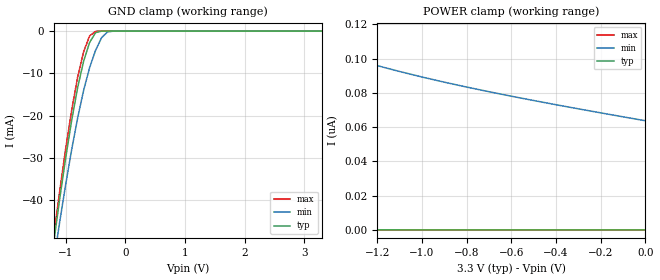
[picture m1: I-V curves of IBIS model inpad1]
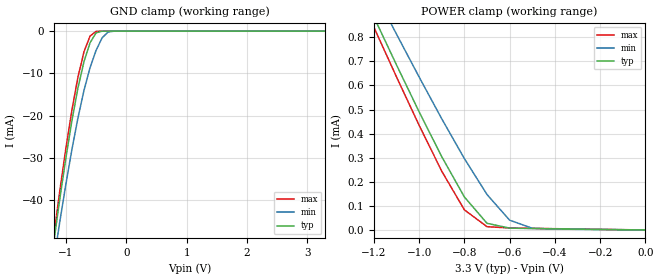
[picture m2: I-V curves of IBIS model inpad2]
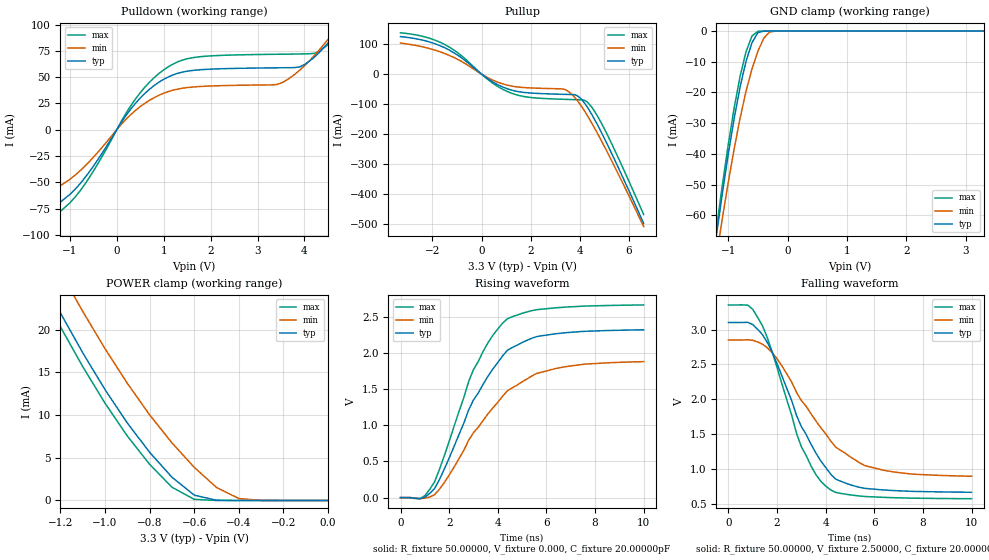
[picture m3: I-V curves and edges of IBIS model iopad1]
| IBIS file 71650da.ibs created by s2ibis2 version 1.2
| North Carolina State University Electronics Research Laboratory  1995
[IBIS ver]   2.1
[File name]   71650da.ibs
[File Rev]   1.2
[Date]   11/10/2004
[Source]   Integrated Device Technology, Inc.
[Notes]   1.Temperatures: typ=25C, min=100C, max=0C
   2.Ramp rates based on 50 ohm load.
   3.The model for the open-drain dta pin does not reflect a
   pulsed pull-up device which aides the output on highz.
[Disclaimer] Integrated Device Technology, Inc. ("IDT") hereby grants the
   user of this IBIS model a non-exclusive, nontransferable
   license to use this IBIS model under the following terms. The
   user is granted this license only to use the IBIS model and is
   not granted rights to sell, copy (except as needed to run the
   IBIS model), rent, lease or sub-license the IBIS model in
   whole or in part, or in modified form to anyone. The User may
   modify the IBIS model to suit its specific applications, but
   rights to derivative works and such modifications shall belong
   to IDT. This IBIS model is provided on an AS IS" basis and IDT
   makes absolutely no warranty with respect to the information
   contained herein. IDT DISCLAIMS AND CUSTOMER WAIVES ALL
   WARRANTIES, EXPRESS AND IMPLIED, INCLUDING WARRANTIES OF
   MERCHANTABILITY AND FITNESS FOR A PARTICULAR PURPOSE. THE
   ENTIRE RISK AS TO QUALITY AND PERFORMANCE IS WITH THE USER
   ACCORDINGLY, IN NO EVENT SHALL IDT BE LIABLE FOR ANY DIRECT OR
   INDIRECT DAMAGES, WHETHER IN CONTRACT OR TORT, INCLUDING ANY
   LOST PROFITS OR OTHER INCIDENTAL, CONSEQUENTIAL, EXEMPLARY, OR
   PUNITIVE DAMAGES ARISING OUT OF THE USE OR APPLICATION OF THE
   IBIS model. Further, IDT reserves the right to make changes
   without notice to any product herein to improve reliability,
   function, or design. IDT does not convey any license under
   patent rights or any other intellectual property rights,
   including those of third parties. IDT is not obligated to
   provide maintenance or support for the licensed IBIS model.
[Copyright]   Copyright 2001, Integrated Device Technology, Inc. all rights
   reserved
|   Component 72v71650
[Component]   72v71650
[Manufacturer]   Integrated Device Technology
[Package]
| DA144
| variable   typ   min   max
R_pkg   51.20m   43.90m   58.40m
L_pkg   4.19nH   3.49nH   4.89nH
C_pkg   0.81pF   0.74pF   0.87pF
[Pin]   signal_name   model_name   R_pin   L_pin   C_pin
143   ode   inpad1
144   resetx   inpad1
2   clk   inpad1
3   foi   inpad1
4   fe_hclk   inpad1
5   wfps   inpad1
6   tms   inpad2
7   tdi   inpad2
8   tdo   iopad1
9   tck   inpad1
10   trstx   inpad2
11   dsx   inpad1
12   csx   inpad1
13   rwx   inpad1
15   a0   inpad1
16   a1   inpad1
17   a2   inpad1
18   a3   inpad1
19   a4   inpad1
20   a5   inpad1
21   a6   inpad1
22   a7   inpad1
23   a8   inpad1
24   a9   inpad1
25   a10   inpad1
26   a11   inpad1
27   a12   inpad1
28   a13   inpad1
29   a14   inpad1
32   dtax   outpad3
35   d15   iopad2
36   d14   iopad2
37   d13   iopad2
38   d12   iopad2
41   d11   iopad2
42   d10   iopad2
43   d9   iopad2
44   d8   iopad2
47   d7   iopad2
48   d6   iopad2
49   d5   iopad2
50   d4   iopad2
53   d3   iopad2
54   d2   iopad2
55   d1   iopad2
56   d0   iopad2
59   rx31   inpad1
60   rx30   inpad1
61   rx29   inpad1
62   rx28   inpad1
63   rx27   inpad1
64   rx26   inpad1
65   rx25   inpad1
66   rx24   inpad1
93   rx23   inpad1
94   rx22   inpad1
95   rx21   inpad1
96   rx20   inpad1
97   rx19   inpad1
98   rx18   inpad1
99   rx17   inpad1
100   rx16   inpad1
101   rx15   inpad1
102   rx14   inpad1
103   rx13   inpad1
104   rx12   inpad1
105   rx11   inpad1
106   rx10   inpad1
107   rx9   inpad1
108   rx8   inpad1
135   rx7   inpad1
136   rx6   inpad1
137   rx5   inpad1
138   rx4   inpad1
139   rx3   inpad1
140   rx2   inpad1
141   rx1   inpad1
142   rx0   inpad1
69   tx31   iopad1
70   tx30   iopad1
71   tx29   iopad1
72   tx28   iopad1
75   tx27   iopad1
76   tx26   iopad1
77   tx25   iopad1
78   tx24   iopad1
81   tx23   iopad1
82   tx22   iopad1
83   tx21   iopad1
84   tx20   iopad1
87   tx19   iopad1
88   tx18   iopad1
89   tx17   iopad1
90   tx16   iopad1
111   tx15   iopad1
112   tx14   iopad1
113   tx13   iopad1
114   tx12   iopad1
117   tx11   iopad1
118   tx10   iopad1
119   tx9   iopad1
120   tx8   iopad1
123   tx7   iopad1
124   tx6   iopad1
125   tx5   iopad1
126   tx4   iopad1
129   tx3   iopad1
130   tx2   iopad1
131   tx1   iopad1
132   tx0   iopad1
110   vdd   POWER
116   vdd   POWER
122   vdd   POWER
128   vdd   POWER
134   vdd   POWER
14   vdd   POWER
33   vdd   POWER
39   vdd   POWER
45   vdd   POWER
51   vdd   POWER
57   vdd   POWER
67   vdd   POWER
73   vdd   POWER
79   vdd   POWER
85   vdd   POWER
91   vdd   POWER
109   vss   GND
115   vss   GND
121   vss   GND
127   vss   GND
133   vss   GND
1   vss   GND
34   vss   GND
40   vss   GND
46   vss   GND
52   vss   GND
58   vss   GND
68   vss   GND
74   vss   GND
80   vss   GND
86   vss   GND
92   vss   GND
| in   in   dummy_model
| oe   oe   dummy_model
[Pin Mapping]  pulldown_ref   pullup_ref   gnd_clamp_ref   power_clamp_ref
143   vss   vdd
144   vss   vdd
2   vss   vdd
3   vss   vdd
4   vss   vdd
5   vss   vdd
6   vss   vdd
7   vss   vdd
8   vss   vdd
9   vss   vdd
10   vss   vdd
11   vss   vdd
12   vss   vdd
13   vss   vdd
15   vss   vdd
16   vss   vdd
17   vss   vdd
18   vss   vdd
19   vss   vdd
20   vss   vdd
21   vss   vdd
22   vss   vdd
23   vss   vdd
24   vss   vdd
25   vss   vdd
26   vss   vdd
27   vss   vdd
28   vss   vdd
29   vss   vdd
32   vss   vdd
35   vss   vdd
36   vss   vdd
37   vss   vdd
38   vss   vdd
41   vss   vdd
42   vss   vdd
43   vss   vdd
44   vss   vdd
47   vss   vdd
48   vss   vdd
49   vss   vdd
50   vss   vdd
53   vss   vdd
54   vss   vdd
55   vss   vdd
56   vss   vdd
59   vss   vdd
60   vss   vdd
61   vss   vdd
62   vss   vdd
63   vss   vdd
64   vss   vdd
65   vss   vdd
66   vss   vdd
93   vss   vdd
94   vss   vdd
95   vss   vdd
96   vss   vdd
97   vss   vdd
98   vss   vdd
99   vss   vdd
100   vss   vdd
101   vss   vdd
102   vss   vdd
103   vss   vdd
104   vss   vdd
105   vss   vdd
106   vss   vdd
107   vss   vdd
108   vss   vdd
135   vss   vdd
136   vss   vdd
137   vss   vdd
138   vss   vdd
139   vss   vdd
140   vss   vdd
141   vss   vdd
142   vss   vdd
69   vss   vdd
70   vss   vdd
71   vss   vdd
72   vss   vdd
75   vss   vdd
76   vss   vdd
77   vss   vdd
78   vss   vdd
81   vss   vdd
82   vss   vdd
83   vss   vdd
84   vss   vdd
87   vss   vdd
88   vss   vdd
89   vss   vdd
90   vss   vdd
111   vss   vdd
112   vss   vdd
113   vss   vdd
114   vss   vdd
117   vss   vdd
118   vss   vdd
119   vss   vdd
120   vss   vdd
123   vss   vdd
124   vss   vdd
125   vss   vdd
126   vss   vdd
129   vss   vdd
130   vss   vdd
131   vss   vdd
132   vss   vdd
110   nc   vdd
116   nc   vdd
122   nc   vdd
128   nc   vdd
134   nc   vdd
14   nc   vdd
33   nc   vdd
39   nc   vdd
45   nc   vdd
51   nc   vdd
57   nc   vdd
67   nc   vdd
73   nc   vdd
79   nc   vdd
85   nc   vdd
91   nc   vdd
109   vss   nc
115   vss   nc
121   vss   nc
127   vss   nc
133   vss   nc
1   vss   nc
34   vss   nc
40   vss   nc
46   vss   nc
52   vss   nc
58   vss   nc
68   vss   nc
74   vss   nc
80   vss   nc
86   vss   nc
92   vss   nc
| Models and submodels in the file (5): inpad1 (Input), inpad2 (Input), iopad1 (3-state), iopad2 (3-state), outpad3 (Open_drain)
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|   Model inpad1
[Model]   inpad1
Model_type   Input
Polarity   Non-Inverting
Vinl =  0.80000V
Vinh =  2.00000V
|Vmeas =  1.50000V
C_comp   5.00000pF   NA   NA
[Temperature Range]   25.00000   100.00000   0.000
[Voltage Range]   3.30000V   3.00000V   3.60000V
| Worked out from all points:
|   GND clamp passes 1 mA (typ) near -0.53 V on its own axis
[GND_clamp]
| voltage   I(typ)   I(min)   I(max)
-3.3V     -310mA     -295.4mA   -315.4mA
-1.2V     -49.78mA   -54.27mA   -48.33mA
-1.1V     -39.5mA    -44.95mA   -37.65mA
-900mV    -21.04mA   -27.95mA   -18.63mA
-800mV    -13.32mA   -20.5mA    -10.85mA
-700mV    -7.09mA    -13.99mA   -4.876mA
-600mV    -2.698mA   -8.653mA   -1.161mA
-500mV    -374.6uA   -4.55mA    -53.22uA
-400mV    -11.83uA   -1.585mA   -1.231uA
-300mV    -285.2nA   -196.8uA   -25.38nA
-200mV    -6.527nA   -10.13uA   -459.3pA
3.3V      26.9pA     70.7nA     2.066pA
[POWER_clamp]
| voltage   I(typ)   I(min)   I(max)
-3.3V     3.879nA    456nA      684.6pA
-3V       2.36nA     327.1nA    413.6pA
-2.7V     1.415nA    242.1nA    246pA
-1.7V     242.2pA    118.8nA    39.53pA
-1.6V     203.7pA    113.3nA    32.78pA
-1.5V     171.8pA    108.3nA    27.21pA
-1.3V     123.7pA    99.68nA    18.83pA
-1.2V     105.8pA    95.94nA    15.74pA
-1V       78.71pA    89.29nA    11.07pA
-800mV    60.2pA     83.42nA    7.956pA
-600mV    47.4pA     78.08nA    5.874pA
0V        26.91pA    63.75nA    2.762pA
|   Model inpad2
[Model]   inpad2
Model_type   Input
Polarity   Non-Inverting
Vinl =  0.80000V
Vinh =  2.00000V
|Vmeas =  1.50000V
C_comp   5.00000pF   NA   NA
[Temperature Range]   26.00000   100.00000   0.000
[Voltage Range]   3.30000V   3.00000V   3.60000V
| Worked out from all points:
|   GND clamp passes 1 mA (typ) near -0.52 V on its own axis
|   POWER clamp passes 1 mA (typ) near -1.26 V on its own axis
[GND_clamp]
| voltage   I(typ)   I(min)   I(max)
-3.3V     -309.8mA   -295.4mA   -315.4mA
-1.2V     -49.84mA   -54.27mA   -48.33mA
-1.1V     -39.57mA   -44.95mA   -37.66mA
-900mV    -21.14mA   -27.95mA   -18.63mA
-800mV    -13.42mA   -20.5mA    -10.85mA
-700mV    -7.183mA   -13.99mA   -4.88mA
-600mV    -2.772mA   -8.654mA   -1.172mA
-500mV    -409.4uA   -4.553mA   -66.79uA
-400mV    -23.35uA   -1.589mA   -14.97uA
-300mV    -10.73uA   -203.7uA   -13.76uA
-200mV    -10.42uA   -17.24uA   -13.74uA
3.3V      29.82pA    2.653uA    -3.476uA
[POWER_clamp]
| voltage   I(typ)   I(min)   I(max)
-3.3V     5.268mA    4.958mA    5.394mA
-1.2V     884.9uA    994.3uA    842.3uA
-1.1V     685.6uA    813.3uA    635.7uA
-1V       490.6uA    635.3uA    434.7uA
-900mV    304.4uA    461.6uA    244uA
-800mV    137uA      296.4uA    83.56uA
-700mV    27.6uA     147.2uA    13.6uA
-600mV    7.666uA    40.58uA    8.253uA
-500mV    5.845uA    7.214uA    6.75uA
0V        29.82pA    63.75nA    2.762pA
|   Model iopad1
[Model]   iopad1
Model_type   3-state
Polarity   Non-Inverting
Enable   Active-High
|Vinl =  0.80000V
|Vinh =  2.00000V
Vmeas =  1.50000V
C_comp   5.00000pF   NA   NA
[Temperature Range]   25.00000   100.00000   0.000
[Voltage Range]   3.30000V   3.00000V   3.60000V
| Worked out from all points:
|   slope of the pulldown table from 0 to 0.495 V, typ, clamps not added: 16.6 ohm
|   slope of the pullup table from 0 to 0.495 V, typ, clamps not added: 17.8 ohm
|   GND clamp passes 1 mA (typ) near -0.51 V on its own axis
|   POWER clamp passes 1 mA (typ) near -0.62 V on its own axis
|   rising waveform, R_fixture 50.00000, V_fixture 0.000, C_fixture 20.00000pF: 20-80 % time 2.08ns typ, 2.41ns min, 1.83ns max; typ from 0 V to 2.32 V
|   falling waveform, R_fixture 50.00000, V_fixture 2.50000, C_fixture 20.00000pF: 20-80 % time 1.86ns typ, 2.29ns min, 1.6ns max; typ from 3.1 V to 0.664 V
[Pulldown]
| voltage   I(typ)   I(min)   I(max)
-3.3V     -98.4mA    -81.6mA    -110.5mA
-1.9V     -86.7mA    -69mA      -97.4mA
-1.3V     -72.39mA   -56.23mA   -81.63mA
-700mV    -46.93mA   -35.66mA   -53.13mA
500mV     30.12mA    21.95mA    35.15mA
1.3V      53.65mA    38.65mA    64.55mA
3.5V      58.91mA    44.27mA    71.8mA
4V        61.97mA    60.76mA    72.13mA
4.3V      72.71mA    74.98mA    74.18mA
4.7V      93.7mA     97.87mA    90.09mA
4.9V      106.9mA    111.1mA    101.7mA
6.6V      332.3mA    305.7mA    332.7mA
[Pullup]
| voltage   I(typ)   I(min)   I(max)
-3.3V     125.2mA    103.6mA    137.8mA
-2.3V     111.4mA    89.05mA    124mA
-1.5V     87.93mA    68.71mA    98.74mA
400mV     -23.23mA   -17.72mA   -26.94mA
1.2V      -52.73mA   -39.41mA   -63mA
3.3V      -67.33mA   -49.39mA   -83.89mA
3.6V      -67.91mA   -61.92mA   -84.61mA
4V        -78.45mA   -99.51mA   -85.44mA
4.2V      -97.4mA    -124.1mA   -87.42mA
4.5V      -136.2mA   -165.3mA   -111.4mA
5.3V      -265.2mA   -289.4mA   -232.6mA
6.6V      -497.9mA   -508.6mA   -468.4mA
[GND_clamp]
| voltage   I(typ)   I(min)   I(max)
-3.3V     -424.5mA   -403.9mA   -432.6mA
-1.2V     -66.92mA   -73.75mA   -64.72mA
-1.1V     -53.15mA   -61.24mA   -50.45mA
-900mV    -28.53mA   -38.43mA   -25.1mA
-800mV    -18.24mA   -28.42mA   -14.76mA
-700mV    -9.879mA   -19.65mA   -6.761mA
-600mV    -3.823mA   -12.36mA   -1.619mA
-500mV    -522.3uA   -6.579mA   -69.89uA
-400mV    -15.84uA   -2.286mA   -1.491uA
-300mV    -368.6nA   -278.7uA   -29.25nA
-200mV    -8.239nA   -14.25uA   -516.1pA
3.3V      29.26pA    12.72uA    2.135pA
[POWER_clamp]
| voltage   I(typ)   I(min)   I(max)
-3.3V     169.2mA    163.5mA    171.9mA
-1.3V     26.89mA    31.6mA     25.32mA
-1.2V     21.93mA    26.74mA    20.31mA
-1.1V     17.28mA    22.12mA    15.66mA
-1V       12.97mA    17.76mA    11.38mA
-900mV    9.066mA    13.71mA    7.542mA
-800mV    5.637mA    10.02mA    4.237mA
-700mV    2.735mA    6.75mA     1.558mA
-600mV    627uA      3.884mA    134.9uA
-500mV    26.21uA    1.53mA     2.445uA
-400mV    585.2nA    230uA      43.52nA
0V        29.28pA    88.51nA    2.883pA
[Ramp]
| variable   typ   min   max
dV/dt_r   1.39320/1.55145n   1.13040/1.90274n   1.59900/1.32996n
dV/dt_f   1.40130/1.59333n   1.10340/2.00863n   1.61178/1.36973n
R_load = 50.00000
[Rising Waveform]
R_fixture = 50.00000
V_fixture = 0.000
C_fixture = 20.00000pF
R_dut = 51.20000m
L_dut = 4.19000nH
C_dut = 0.81000pF
| time   V(typ)   V(min)   V(max)
0s        0V         0V         0V
800ps     -15.33mV   -14.76mV   -14.41mV
1.4ns     123.7mV    40.45mV    217mV
2ns       545.2mV    310.4mV    777mV
3ns       1.348V     895.9mV    1.767V
3.8ns     1.776V     1.239V     2.242V
4.4ns     2.034V     1.476V     2.47V
5.6ns     2.223V     1.714V     2.595V
6.4ns     2.263V     1.782V     2.62V
10ns      2.316V     1.877V     2.66V
[Falling Waveform]
R_fixture = 50.00000
V_fixture = 2.50000
C_fixture = 20.00000pF
R_dut = 51.20000m
L_dut = 4.19000nH
C_dut = 0.81000pF
| time   V(typ)   V(min)   V(max)
0s        3.103V     2.852V     3.355V
800ps     3.105V     2.855V     3.352V
1.4ns     2.929V     2.791V     3.056V
2ns       2.51V      2.582V     2.454V
3ns       1.606V     1.981V     1.316V
3.6ns     1.225V     1.687V     915.6mV
4ns       1.019V     1.503V     753mV
4.4ns     855.4mV    1.315V     662.5mV
5.6ns     719.8mV    1.048V     602.8mV
10ns      663.6mV    894.1mV    571mV
